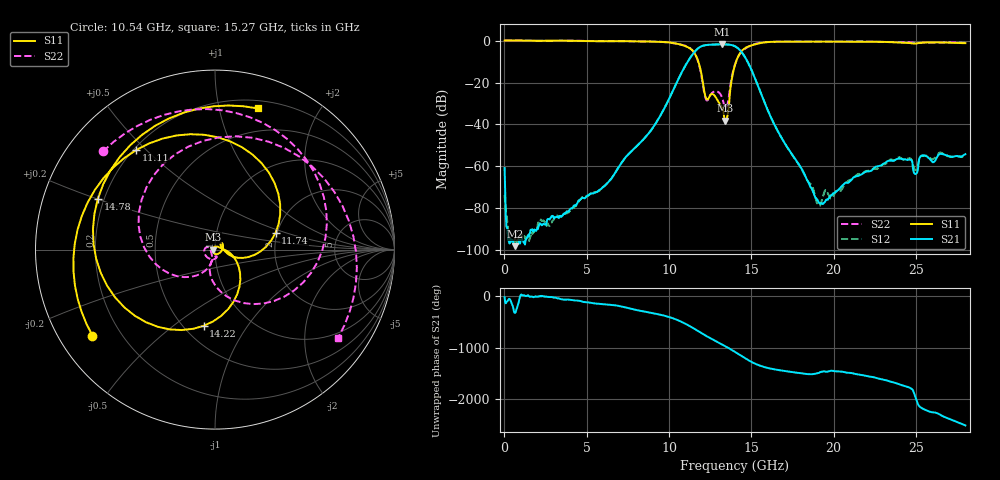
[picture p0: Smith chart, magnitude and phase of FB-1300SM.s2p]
! MARKI MICROWAVE INC.
! Email:  info@markimicrowave.com  Phone:  408-778-4200
! Model Number:  FB-1300SM  Date:  02/11
! Filename:		FB-1300SM.S2P  Version: 1.0
! Description:  2-port S-parameter data for Surface Mount Band Pass Filter FB-1300SM, measured in a connectorized fixture
! Frequency Range: 	10 MHz to 28 GHz
! Measurements:		S11, S21, S12, S22
# Hz S  dB  R 50
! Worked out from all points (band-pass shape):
!   748 points, 10 MHz to 28.01 GHz, reference 50 ohm
!   highest |S21| = -1.79 dB at 13.24 GHz (marker M1); lowest = -98.1 dB at 647.3 MHz (marker M2)
!   |S21| within 3 dB of the highest: 11.62 GHz to 14.34 GHz (2.722 GHz wide, 21 % of centre)
!   lowest |S11| = -38.2 dB at 13.43 GHz (marker M3), VSWR 1.02, Z = 48.8 + j0.0351 ohm
!   |S11| at or under -10 dB: 11.78 GHz to 14.08 GHz (2.294 GHz wide, 17.7 % of centre)
!   |S22| runs from -32.2 to 0.1 dB; largest |S21 - S12| = 0.00074
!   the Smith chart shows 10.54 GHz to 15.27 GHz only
!   S11 on the Smith chart (normalised r, x): 10.54 GHz: 0.10, -0.31; 11.11 GHz: 0.21, +0.47; 11.74 GHz: 1.96, +0.42; 14.22 GHz: 0.62, -0.65; 14.78 GHz: 0.18, +0.20; 15.27 GHz: 0.27, +1.31
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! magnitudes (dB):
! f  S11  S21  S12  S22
! 10 MHz  0.0  -60.8  -73.7  0.1
! 197.4 MHz  0.0  -92.3  -88.7  0.1
! 647.3 MHz  0.1  -98.1  -94.0  0.1
! 4.696 GHz  -0.2  -75.2  -74.9  -0.2
! 6.27 GHz  -0.3  -67.9  -67.9  -0.2
! 9.344 GHz  -0.6  -37.6  -37.6  -0.5
! 10.54 GHz  -1.6  -18.8  -18.8  -1.6
! 11.11 GHz  -3.0  -10.5  -10.5  -2.8
! 11.74 GHz  -9.1  -3.8  -3.8  -9.4
! 12.27 GHz  -27.7  -2.1  -2.1  -28.3
! 13.24 GHz  -32.2  -1.8  -1.8  -27.6
! 13.43 GHz  -38.2  -1.8  -1.8  -32.2
! 14.03 GHz  -11.1  -2.8  -2.8  -10.9
! 14.22 GHz  -7.3  -3.8  -3.8  -7.5
! 14.78 GHz  -3.0  -10.1  -10.1  -3.1
! 15.27 GHz  -1.7  -18.8  -18.8  -1.5
! 18.68 GHz  -0.5  -70.8  -69.2  -0.5
! 19.13 GHz  -0.5  -77.5  -78.9  -0.5
! 23.36 GHz  -0.7  -57.3  -57.3  -0.7
! 24.98 GHz  -1.4  -63.6  -61.6  -1.1
! 25.39 GHz  -1.0  -54.8  -55.0  -1.1
! 28.01 GHz  -1.2  -54.2  -54.8  -1.1
